| / 7\'7   Xilinx CoolRunner XPLA3 I/O Buffer IBIS File
| \ \   Xilinx Inc.
| / /   2100 Logic Drive
| \_\/.\   San Jose,   CA 95124
[IBIS ver]   2.1
[File name]   xpla3.ibs
[File Rev]   1.1
[Date]   March 30, 2000
[Source]   Spice netlist
[Notes]   - Control flag setting:
   SLW=0 - fast slew rate
   SEW=1 - slow slew rate
   - Created by Joey Jia x4437
[Disclaimer] The data in this model is derived from SPICE simulations using
   modeling information extracted from the target process. While
   a great deal of care has been take to provide information that
   is accurate, this model is considered preliminary as it has
   not been verified by actual silicon measurement. Treat the
   data in this model as preliminary until actual silicon
   verification is performed.
[Copyright]   Xilinx Inc. All right reserved
|   Component XCR3064XL_CP56[SLW=0]
[Component]   XCR3064XL_CP56[SLW=0]
[Manufacturer]   Xilinx Inc.
[Package]
| variable   typ   min   max
R_pkg   89.000m   75.000m   103.000m
L_pkg   1.850nH   1.500nH   2.200nH
C_pkg   0.350pF   0.300pF   0.400pF
[Pin]  signal_name   model_name   R_pin   L_pin   C_pin
io   PIN   IO_00   NA   NA   NA
| End [Component] XCR3064XL_CP56[SLW=0]
|   Component XCR3064XL_CP56[SLW=1]
[Component]   XCR3064XL_CP56[SLW=1]
[Manufacturer]   Xilinx Inc.
[Package]
| variable   typ   min   max
R_pkg   89.000m   75.000m   103.000m
L_pkg   1.850nH   1.500nH   2.200nH
C_pkg   0.350pF   0.300pF   0.400pF
[Pin]  signal_name   model_name   R_pin   L_pin   C_pin
io   PIN   IO_01   NA   NA   NA
| End [Component] XCR3064XL_CP56[SLW=1]
|   Component XCR3064XL_CS48[SLW=0]
[Component]   XCR3064XL_CS48[SLW=0]
[Manufacturer]   Xilinx Inc.
[Package]
| variable   typ   min   max
R_pkg   112.000m   98.000m   126.000m
L_pkg   2.100nH   1.800nH   2.400nH
C_pkg   0.250pF   0.200pF   0.300pF
[Pin]  signal_name   model_name   R_pin   L_pin   C_pin
io   PIN   IO_00   NA   NA   NA
| End [Component] XCR3064XL_CS48[SLW=0]
|   Component XCR3064XL_CS48[SLW=1]
[Component]   XCR3064XL_CS48[SLW=1]
[Manufacturer]   Xilinx Inc.
[Package]
| variable   typ   min   max
R_pkg   112.000m   98.000m   126.000m
L_pkg   2.100nH   1.800nH   2.400nH
C_pkg   0.250pF   0.200pF   0.300pF
[Pin]  signal_name   model_name   R_pin   L_pin   C_pin
io   PIN   IO_01   NA   NA   NA
| End [Component] XCR3064XL_CS48[SLW=1]
|   Component XCR3064XL_VQ44[SLW=0]
[Component]   XCR3064XL_VQ44[SLW=0]
[Manufacturer]   Xilinx Inc.
[Package]
| variable   typ   min   max
R_pkg   57.000m   54.000m   60.000m
L_pkg   2.250nH   2.100nH   2.400nH
C_pkg   0.300pF   0.300pF   0.300pF
[Pin]  signal_name   model_name   R_pin   L_pin   C_pin
io   PIN   IO_00   NA   NA   NA
| End [Component] XCR3064XL_VQ44[SLW=0]
|   Component XCR3064XL_VQ44[SLW=1]
[Component]   XCR3064XL_VQ44[SLW=1]
[Manufacturer]   Xilinx Inc.
[Package]
| variable   typ   min   max
R_pkg   57.000m   54.000m   60.000m
L_pkg   2.250nH   2.100nH   2.400nH
C_pkg   0.300pF   0.300pF   0.300pF
[Pin]  signal_name   model_name   R_pin   L_pin   C_pin
io   PIN   IO_01   NA   NA   NA
| End [Component] XCR3064XL_VQ44[SLW=1]
|   Component XCR3064XL_VQ100[SLW=0]
[Component]   XCR3064XL_VQ100[SLW=0]
[Manufacturer]   Xilinx Inc.
[Package]
| variable   typ   min   max
R_pkg   101.500m   98.000m   105.000m
L_pkg   5.200nH   4.700nH   5.700nH
C_pkg   0.550pF   0.400pF   0.700pF
[Pin]  signal_name   model_name   R_pin   L_pin   C_pin
io   PIN   IO_00   NA   NA   NA
| End [Component] XCR3064XL_VQ100[SLW=0]
|   Component XCR3064XL_VQ100[SLW=1]
[Component]   XCR3064XL_VQ100[SLW=1]
[Manufacturer]   Xilinx Inc.
[Package]
| variable   typ   min   max
R_pkg   101.500m   98.000m   105.000m
L_pkg   5.200nH   4.700nH   5.700nH
C_pkg   0.550pF   0.400pF   0.700pF
[Pin]  signal_name   model_name   R_pin   L_pin   C_pin
io   PIN   IO_01   NA   NA   NA
| End [Component] XCR3064XL_VQ100[SLW=1]
|   Component XCR3128XL_CS144[SLW=0]
[Component]   XCR3128XL_CS144[SLW=0]
[Manufacturer]   Xilinx Inc.
[Package]
| variable   typ   min   max
R_pkg   109.500m   76.000m   143.000m
L_pkg   2.250nH   1.500nH   3.000nH
C_pkg   0.250pF   0.200pF   0.300pF
[Pin]  signal_name   model_name   R_pin   L_pin   C_pin
io   PIN   IO_00   NA   NA   NA
| End [Component] XCR3128XL_CS144[SLW=0]
|   Component XCR3128XL_CS144[SLW=1]
[Component]   XCR3128XL_CS144[SLW=1]
[Manufacturer]   Xilinx Inc.
[Package]
| variable   typ   min   max
R_pkg   109.500m   76.000m   143.000m
L_pkg   2.250nH   1.500nH   3.000nH
C_pkg   0.250pF   0.200pF   0.300pF
[Pin]  signal_name   model_name   R_pin   L_pin   C_pin
io   PIN   IO_01   NA   NA   NA
| End [Component] XCR3128XL_CS144[SLW=1]
|   Component XCR3128XL_TQ144[SLW=0]
[Component]   XCR3128XL_TQ144[SLW=0]
[Manufacturer]   Xilinx Inc.
[Package]
| variable   typ   min   max
R_pkg   123.500m   117.000m   130.000m
L_pkg   7.950nH   7.100nH   8.800nH
C_pkg   1.000pF   0.800pF   1.200pF
[Pin]  signal_name   model_name   R_pin   L_pin   C_pin
io   PIN   IO_00   NA   NA   NA
| End [Component] XCR3128XL_TQ144[SLW=0]
|   Component XCR3128XL_TQ144[SLW=1]
[Component]   XCR3128XL_TQ144[SLW=1]
[Manufacturer]   Xilinx Inc.
[Package]
| variable   typ   min   max
R_pkg   123.500m   117.000m   130.000m
L_pkg   7.950nH   7.100nH   8.800nH
C_pkg   1.000pF   0.800pF   1.200pF
[Pin]  signal_name   model_name   R_pin   L_pin   C_pin
io   PIN   IO_01   NA   NA   NA
| End [Component] XCR3128XL_TQ144[SLW=1]
|   Component XCR3128XL_VQ100[SLW=0]
[Component]   XCR3128XL_VQ100[SLW=0]
[Manufacturer]   Xilinx Inc.
[Package]
| variable   typ   min   max
R_pkg   101.500m   98.000m   105.000m
L_pkg   5.200nH   4.700nH   5.700nH
C_pkg   0.550pF   0.400pF   0.700pF
[Pin]  signal_name   model_name   R_pin   L_pin   C_pin
io   PIN   IO_00   NA   NA   NA
| End [Component] XCR3128XL_VQ100[SLW=0]
|   Component XCR3128XL_VQ100[SLW=1]
[Component]   XCR3128XL_VQ100[SLW=1]
[Manufacturer]   Xilinx Inc.
[Package]
| variable   typ   min   max
R_pkg   101.500m   98.000m   105.000m
L_pkg   5.200nH   4.700nH   5.700nH
C_pkg   0.550pF   0.400pF   0.700pF
[Pin]  signal_name   model_name   R_pin   L_pin   C_pin
io   PIN   IO_01   NA   NA   NA
| End [Component] XCR3128XL_VQ100[SLW=1]
|   Component XCR3256XL_CS280[SLW=0]
[Component]   XCR3256XL_CS280[SLW=0]
[Manufacturer]   Xilinx Inc.
[Package]
| variable   typ   min   max
R_pkg   259.500m   148.000m   371.000m
L_pkg   5.800nH   2.700nH   8.900nH
C_pkg   0.500pF   0.200pF   0.800pF
[Pin]  signal_name   model_name   R_pin   L_pin   C_pin
io   PIN   IO_00   NA   NA   NA
| End [Component] XCR3256XL_CS280[SLW=0]
|   Component XCR3256XL_CS280[SLW=1]
[Component]   XCR3256XL_CS280[SLW=1]
[Manufacturer]   Xilinx Inc.
[Package]
| variable   typ   min   max
R_pkg   259.500m   148.000m   371.000m
L_pkg   5.800nH   2.700nH   8.900nH
C_pkg   0.500pF   0.200pF   0.800pF
[Pin]  signal_name   model_name   R_pin   L_pin   C_pin
io   PIN   IO_01   NA   NA   NA
| End [Component] XCR3256XL_CS280[SLW=1]
|   Component XCR3256XL_PQ208[SLW=0]
[Component]   XCR3256XL_PQ208[SLW=0]
[Manufacturer]   Xilinx Inc.
[Package]
| variable   typ   min   max
R_pkg   195.500m   195.000m   196.000m
L_pkg   14.200nH   12.500nH   15.900nH
C_pkg   1.800pF   1.600pF   2.000pF
[Pin]  signal_name   model_name   R_pin   L_pin   C_pin
io   PIN   IO_00   NA   NA   NA
| End [Component] XCR3256XL_PQ208[SLW=0]
|   Component XCR3256XL_PQ208[SLW=1]
[Component]   XCR3256XL_PQ208[SLW=1]
[Manufacturer]   Xilinx Inc.
[Package]
| variable   typ   min   max
R_pkg   195.500m   195.000m   196.000m
L_pkg   14.200nH   12.500nH   15.900nH
C_pkg   1.800pF   1.600pF   2.000pF
[Pin]  signal_name   model_name   R_pin   L_pin   C_pin
io   PIN   IO_01   NA   NA   NA
| End [Component] XCR3256XL_PQ208[SLW=1]
|   Component XCR3256XL_TQ144[SLW=0]
[Component]   XCR3256XL_TQ144[SLW=0]
[Manufacturer]   Xilinx Inc.
[Package]
| variable   typ   min   max
R_pkg   123.500m   117.000m   130.000m
L_pkg   7.950nH   7.100nH   8.800nH
C_pkg   1.000pF   0.800pF   1.200pF
[Pin]  signal_name   model_name   R_pin   L_pin   C_pin
io   PIN   IO_00   NA   NA   NA
| End [Component] XCR3256XL_TQ144[SLW=0]
|   Component XCR3256XL_TQ144[SLW=1]
[Component]   XCR3256XL_TQ144[SLW=1]
[Manufacturer]   Xilinx Inc.
[Package]
| variable   typ   min   max
R_pkg   123.500m   117.000m   130.000m
L_pkg   7.950nH   7.100nH   8.800nH
C_pkg   1.000pF   0.800pF   1.200pF
[Pin]  signal_name   model_name   R_pin   L_pin   C_pin
io   PIN   IO_01   NA   NA   NA
| End [Component] XCR3256XL_TQ144[SLW=1]
| Models and submodels in the file (2): IO_00 (I/O), IO_01 (I/O)
